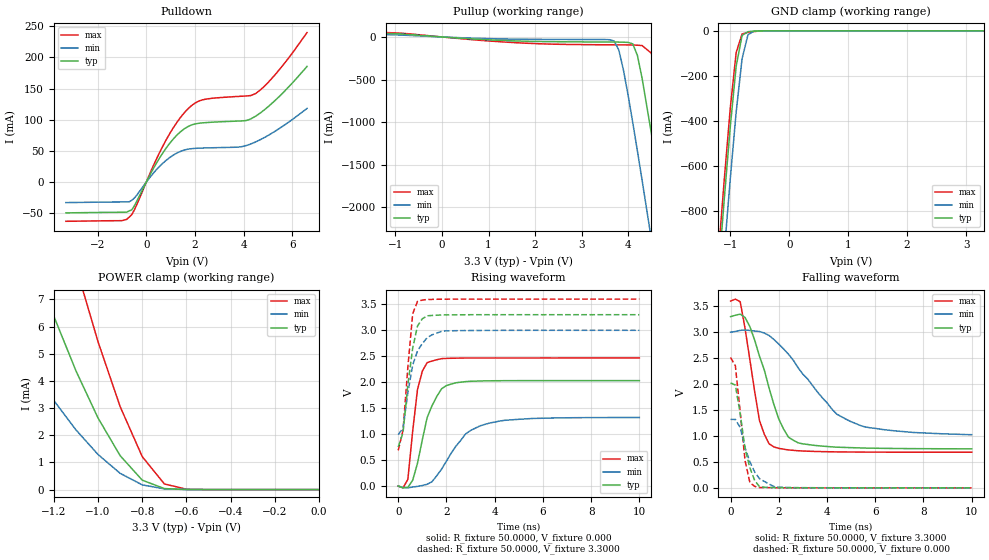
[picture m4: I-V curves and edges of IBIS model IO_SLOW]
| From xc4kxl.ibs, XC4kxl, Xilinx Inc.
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|   Model IO_SLOW
[Model]   IO_SLOW
Model_type   I/O
Polarity   Non-Inverting
Enable   Active-Low
Vinl = 0.8V
Vinh = 2.0V
Vmeas =   1.6500V
Cref =  50.0000pF
Rref =   1.0000M
Vref =  0.000V
C_comp   7.0000pF   6.0000pF   8.0000pF
[Temperature Range]   27.0000   100.0000   0.000
[Voltage Range]   3.3000V   3.0000V   3.6000V
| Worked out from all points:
|   slope of the pulldown table from 0 to 0.495 V, typ, clamps not added: 13.9 ohm
|   slope of the pullup table from 0 to 0.495 V, typ, clamps not added: 27.1 ohm
|   GND clamp passes 1 mA (typ) near -0.58 V on its own axis
|   POWER clamp passes 1 mA (typ) near -0.87 V on its own axis
|   rising waveform, R_fixture 50.0000, V_fixture 0.000: 20-80 % time 708ps typ, 1.25ns min, 387ps max; typ from 0 V to 2.03 V
|   rising waveform, R_fixture 50.0000, V_fixture 3.3000: 20-80 % time 413ps typ, 515ps min, 309ps max; typ from 0.751 V to 3.3 V
|   falling waveform, R_fixture 50.0000, V_fixture 3.3000: 20-80 % time 1.03ns typ, 2.06ns min, 600ps max; typ from 3.3 V to 0.752 V
|   falling waveform, R_fixture 50.0000, V_fixture 0.000: 20-80 % time 461ps typ, 610ps min, 335ps max; typ from 2.02 V to 0 V
[Pulldown]
| voltage   I(typ)   I(min)   I(max)
-3.3V     -49.3mA    -32.8mA    -62.8mA
-800mV    -48.11mA   -31.6mA    -59.6mA
-500mV    -38.84mA   -25.82mA   -45.39mA
300mV     22.39mA    14.76mA    27.1mA
800mV     53.74mA    34.43mA    66.56mA
1.3V      76.97mA    47.48mA    98.21mA
1.7V      88.86mA    52.78mA    117.1mA
2.3V      95.03mA    54.68mA    131.9mA
3.8V      98.02mA    56.26mA    137.5mA
4.5V      106mA      64.68mA    142.4mA
5.3V      131.4mA    81.93mA    172.8mA
6.6V      185.5mA    118.2mA    239.9mA
[Pullup]
| voltage   I(typ)   I(min)   I(max)
-3.3V     63.98mA    45.77mA    74.9mA
3.7V      -59.9mA    -48.13mA   -92.59mA
3.8V      -60.3mA    -155.1mA   -92.88mA
3.9V      -61.55mA   -391.7mA   -93.16mA
4.1V      -81.44mA   -1.009A    -94.6mA
4.2V      -218.1mA   -1.343A    -97.2mA
4.3V      -487mA     -1.684A    -101mA
4.5V      -1.135A    -2.381A    -191.2mA
4.7V      -1.825A    -3.088A    -749.8mA
4.9V      -2.532A    -3.801A    -1.425A
5.1V      -3.246A    -4.519A    -2.126A
6.6V      -8.69A     -9.964A    -7.553A
[GND_clamp]
| voltage   I(typ)   I(min)   I(max)
-3.3V     -8.626A    -8.837A    -8.551A
-1.2V     -1.073A    -1.312A    -987.3mA
-1.1V     -740.8mA   -978.2mA   -654.8mA
-1V       -426mA     -657.1mA   -343.9mA
-900mV    -157.2mA   -360.9mA   -96.62mA
-800mV    -20.77mA   -124.4mA   -14.17mA
-700mV    -3.846mA   -17.61mA   -6.82mA
-600mV    -1.246mA   -1.662mA   -3.283mA
-300mV    -276.3nA   -435.5nA   -2.755uA
3.3V      151.6pA    7.389nA    160.3pA
[POWER_clamp]
| voltage   I(typ)   I(min)   I(max)
-3.3V     75.42mA    47.28mA    100.2mA
-1.5V     13.67mA    7.363mA    21.72mA
-1.4V     11.06mA    5.873mA    18.06mA
-1.3V     8.626mA    4.508mA    14.56mA
-1.2V     6.385mA    3.279mA    11.27mA
-1.1V     4.373mA    2.199mA    8.21mA
-1V       2.636mA    1.293mA    5.443mA
-900mV    1.25mA     599.1uA    3.055mA
-800mV    347.4uA    174.4uA    1.214mA
-700mV    37.68uA    27.06uA    209.3uA
-600mV    2.828uA    3.397uA    13.73uA
0V        151.5pA    186pA      177.1pA
[Ramp]
| variable   typ   min   max
dV/dt_r   1.1778/0.6374n   0.7470/1.2967n   1.4802/0.3854n
dV/dt_f   1.5286/0.9702n   1.1850/2.1524n   1.7479/0.5879n
R_load = 50.0000
[Rising Waveform]
R_fixture = 50.0000
V_fixture = 0.000
| time   V(typ)   V(min)   V(max)
0s        0V         0V         0V
200ps     -34.28mV   -25.59mV   -34.33mV
400ps     -24.33mV   -34.12mV   129.9mV
600ps     111.5mV    -18.21mV   1.058V
800ps     439mV      -6.026mV   1.859V
1.2ns     1.32V      35.15mV    2.377V
1.8ns     1.874V     328.4mV    2.453V
2.8ns     2.012V     1.007V     2.465V
3.4ns     2.023V     1.16V      2.466V
10ns      2.03V      1.32V      2.467V
[Rising Waveform]
R_fixture = 50.0000
V_fixture = 3.3000
V_fixture_min = 3.0000
V_fixture_max = 3.6000
| time   V(typ)   V(min)   V(max)
0s        750.6mV    990.1mV    686.6mV
200ps     1.03V      1.117V     1.071V
400ps     1.945V     1.795V     2.29V
600ps     2.655V     2.327V     3.318V
800ps     3.082V     2.603V     3.556V
1ns       3.221V     2.744V     3.58V
1.2ns     3.278V     2.856V     3.592V
1.6ns     3.289V     2.946V     3.596V
2ns       3.296V     2.989V     3.598V
10ns      3.299V     2.999V     3.599V
[Falling Waveform]
R_fixture = 50.0000
V_fixture = 3.3000
V_fixture_min = 3.0000
V_fixture_max = 3.6000
| time   V(typ)   V(min)   V(max)
0s        3.3V       3V         3.6V
400ps     3.349V     3.035V     3.588V
800ps     3.11V      3.034V     2.474V
1.2ns     2.538V     3.014V     1.296V
1.8ns     1.603V     2.86V      789mV
2.2ns     1.133V     2.678V     746.1mV
2.6ns     918.3mV    2.463V     723.4mV
4.4ns     784.1mV    1.422V     693.3mV
5ns       775.2mV    1.276V     691.2mV
10ns      752.3mV    1.025V     686.9mV
[Falling Waveform]
R_fixture = 50.0000
V_fixture = 0.000
| time   V(typ)   V(min)   V(max)
0s        2.025V     1.32V      2.513V
200ps     1.98V      1.319V     2.352V
400ps     1.428V     1.163V     1.46V
600ps     766.4mV    776.4mV    527.9mV
800ps     389.2mV    503.9mV    104.6mV
1ns       142.7mV    307mV      27.72mV
1.2ns     23.92mV    176.7mV    7.611mV
1.8ns     5.596mV    26.32mV    2.983mV
2ns       4.084mV    14.64mV    2.244mV
10ns      225.2uV    532.6uV    159.7uV
